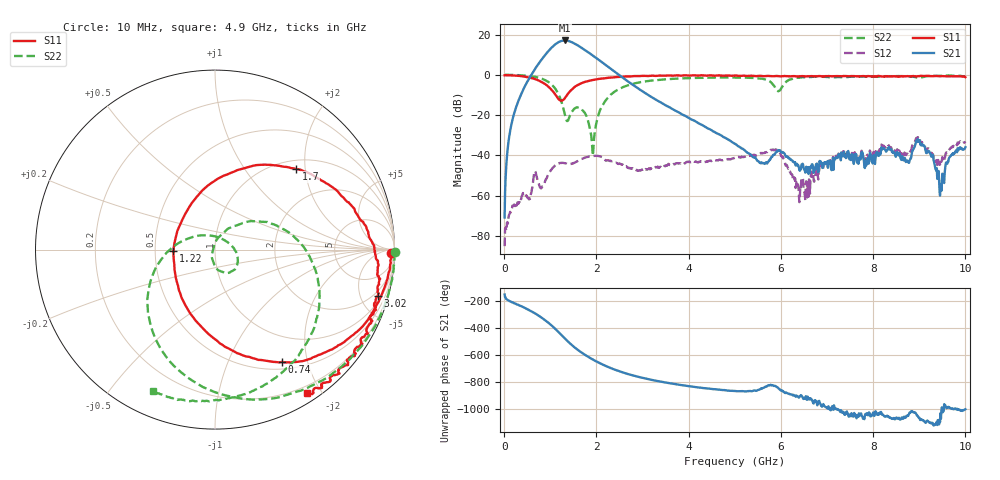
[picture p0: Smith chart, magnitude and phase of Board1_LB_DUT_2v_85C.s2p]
! Created Tue May 27 16:26:11 2025
# hz S ma R 50
! 2 Port Network Data from SP1.SP block
! freq  magS11  angS11  magS21  angS21  magS12  angS12  magS22  angS22
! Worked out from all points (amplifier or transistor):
!   1000 points, 10 MHz to 10 GHz, reference 50 ohm
!   highest |S21| = 17.1 dB at 1.31 GHz (marker M1)
!   |S21| within 3 dB of that: 1.055 GHz to 1.636 GHz (580.9 MHz wide, 43.2 % of centre)
!   unconditionally stable (mu >= 1): 58.45 MHz to 62.47 MHz; 89.7 MHz to 103.3 MHz; 116 MHz to end of sweep
!   at 1.67 GHz: K = 7.99, MAG = 15.7 dB, |S12| = -41.9 dB
!   at 5.01 GHz: K = 46.50, MAG = -16.3 dB, |S12| = -41.2 dB
!   at 10 GHz: K = 55.09, MAG = -21.9 dB, |S12| = -33.1 dB
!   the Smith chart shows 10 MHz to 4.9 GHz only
!   S11 on the Smith chart (normalised r, x): 10 MHz: 54, -45; 740 MHz: 0.60, -1.60; 1.22 GHz: 0.62, -0.01; 1.7 GHz: 1.18, +1.79; 3.02 GHz: 1.49, -6.82; 4.9 GHz: 0.11, -1.82
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1e7  0.9784 -1.1  0.0002836 -153.5  5.504e-05 159.8  1.005 -0.8
1.9e8  0.9673 -12.9  0.08522 148.3  0.0005473 78.7  0.9955 -16.9
7.4e8  0.7286 -59.2  1.844 52.0  0.002134 60.4  0.8566 -77.0
9e8  0.5769 -79.4  3.24 14.1  0.002515 109.8  0.73 -101.8
1.04e9  0.4094 -105.4  4.898 -25.2  0.00467 99.9  0.5597 -129.3
1.13e9  0.3017 -131.9  6.012 -53.9  0.005928 86.1  0.4157 -151.4
1.22e9  0.2318 -177.6  6.841 -84.6  0.006457 71.9  0.253 -179.5
1.31e9  0.2574 130.7  7.179 -115.8  0.006417 61.3  0.111 134.2
1.47e9  0.4362 78.4  6.472 -167.2  0.006232 57.8  0.1218 -10.4
1.68e9  0.6224 46.8  4.703 137.6  0.008097 50.0  0.141 -66.4
1.7e9  0.6378 44.8  4.547 133.0  0.00827 48.8  0.1321 -70.8
1.9e9  0.7381 28.4  3.164 91.1  0.009551 29.9  0.02201 -132.0
2.11e9  0.8096 16.3  2.114 53.8  0.009213 5.9  0.1562 53.8
2.48e9  0.888 0.2  1.022 1.8  0.006078 -6.0  0.4383 10.6
3.02e9  0.942 -15.9  0.3767 -50.2  0.004473 5.8  0.6774 -32.4
3.34e9  0.9523 -24.3  0.2232 -72.9  0.00499 8.6  0.7504 -51.4
4.9e9  0.9513 -57.4  0.02302 -144.1  0.007978 -6.9  0.8609 -113.8
5.01e9  0.9687 -59.5  0.0192 -145.6  0.008731 -10.6  0.8618 -117.7
6.67e9  0.9323 -90.7  0.005944 149.5  0.003734 143.3  0.8899 -149.9
8.34e9  0.9127 -135.5  0.01588 21.0  0.01772 31.7  0.9205 172.7
9.49e9  0.9308 -167.7  0.002104 93.5  0.007532 68.3  0.9532 164.3
1e10  0.8756 177.9  0.01585 79.7  0.02216 71.6  0.9146 163.5
